FUNCTION_BLOCK FB_DirectControl EXTENDS FB_AsyncServiceResultClass
VAR
	_ipClient 	: I_ScsmClientClass;	
	_ipCtrl 	: I_AcsiCommonControllableDataClass;(* interface pointer to controllable data object *)

	_ctlVal		: U_AcsiCtlVal;
	_operTm 	: T_UtcTime;
	_origin		: ST_AcsiOriginator := ( orCat := E_AcsiOrCategory.StationControl, orIdent := [16#BE,16#CF,16#61,16#85] );
	_ctlNum		: USINT;
	_bTest 		: BOOL;
	_eCheck		: E_AcsiCheck := E_AcsiCheck.NoCheck; 	

	_nInvokeID 	: UDINT;
	_ipResult 	: I_AsyncServiceResultClass;

	_tmpCtlVal	: U_AcsiCtlVal;
	_bMxVal		: BOOL;
	state 		: UDINT;
END_VAR

METHOD APC : BOOL
VAR_INPUT
	ipClient 	: I_ScsmClientClass;	
	ipCtrl 		: I_AcsiCommonControllableDataClass;
	ctlVal		: REAL;
END_VAR
VAR_OUTPUT
	ipResult 	: I_AsyncServiceResultClass;
END_VAR
_tmpCtlVal.APC.f:= ctlVal;
APC:= Request(ipClient:=ipClient, ipCtrl:=ipCtrl, ctlVal:=_tmpCtlVal, bMxVal:=TRUE, ipResult=>ipResult);
END_METHOD

METHOD BAC : BOOL
VAR_INPUT
	ipClient 	: I_ScsmClientClass;	
	ipCtrl 		: I_AcsiCommonControllableDataClass;
	ctlVal		: E_AcsiTcmd;
END_VAR
VAR_OUTPUT
	ipResult 	: I_AsyncServiceResultClass;
END_VAR
_tmpCtlVal.BAC:= ctlVal;
BAC:= Request(ipClient:=ipClient, ipCtrl:=ipCtrl, ctlVal:=_tmpCtlVal, bMxVal:=TRUE, ipResult=>ipResult);
END_METHOD

METHOD BSC : BOOL
VAR_INPUT
	ipClient 	: I_ScsmClientClass;	
	ipCtrl 		: I_AcsiCommonControllableDataClass;
	ctlVal		: E_AcsiTcmd;
END_VAR
VAR_OUTPUT
	ipResult 	: I_AsyncServiceResultClass;
END_VAR
_tmpCtlVal.BSC:= ctlVal;
BSC:= Request(ipClient:=ipClient, ipCtrl:=ipCtrl, ctlVal:=_tmpCtlVal, bMxVal:=FALSE, ipResult=>ipResult);
END_METHOD

PROPERTY bTest : BOOL
SET
_bTest:= bTest;
END_SET
END_PROPERTY

METHOD Clear
VAR_INPUT
	ipReason : I_ServiceErrorClass;
END_VAR
IF SUPER^.IsBusy() THEN
	SUPER^.SetAborted(ipReason:=ipReason);
END_IF
state:= 0;
END_METHOD

METHOD DPC : BOOL
VAR_INPUT
	ipClient 	: I_ScsmClientClass;	
	ipCtrl 		: I_AcsiCommonControllableDataClass;
	ctlVal		: BOOL;
END_VAR
VAR_OUTPUT
	ipResult 	: I_AsyncServiceResultClass;
END_VAR
_tmpCtlVal.DPC:= ctlVal;
DPC:= Request(ipClient:=ipClient, ipCtrl:=ipCtrl, ctlVal:=_tmpCtlVal, bMxVal:=FALSE, ipResult=>ipResult);
END_METHOD

PROPERTY eCheck : E_AcsiCheck
SET
_eCheck:= eCheck;
END_SET
END_PROPERTY

METHOD ENC_Mod : BOOL
VAR_INPUT
	ipClient 	: I_ScsmClientClass;	
	ipCtrl 		: I_AcsiCommonControllableDataClass;
	ctlVal		: E_AcsiMod;
END_VAR
VAR_OUTPUT
	ipResult 	: I_AsyncServiceResultClass;
END_VAR
_tmpCtlVal.ENC.Mode:= ctlVal;
ENC_Mod:= Request(ipClient:=ipClient, ipCtrl:=ipCtrl, ctlVal:=_tmpCtlVal, bMxVal:=FALSE, ipResult=>ipResult);
END_METHOD

METHOD Execute : BOOL
CASE state OF
	0:RETURN;(* idle state *)

	(*--------------------- Verify status (optional) -----------------------------------*)
	1: (* Read control status information e.g.: "IEDLD1/CSWI1.ST.Pos" (stVal, q, t, ...) *)
		state:= SEL(_ipClient.GetDataValuesReq(ipData:=_ipCtrl, eFC:=SEL(_bMxVal, E_AcsiFc.ST_, E_AcsiFc.MX), hUser:=0, ipSink:=0, nInvokeID=>_nInvokeID, ipResult=>_ipResult), 100, 2); 
	2:
		IF _ipResult <> 0 THEN
			_ipResult.Execute();
			IF NOT _ipResult.IsBusy() THEN
				state:= SEL(_ipResult.IsCompleted(), 100, 10);
			END_IF
		END_IF
		
	(*--------------------- Verify config (optional) ------------------------------------*)
	10: (* Read control configuration e.g.: "IEDLD1/CSWI1.CF.Pos" (ctlModel, pulseConfig, ...) *)
		state:= SEL(_ipClient.GetDataValuesReq(ipData:=_ipCtrl, eFC:=E_AcsiFc.CF, hUser:=0, ipSink:=0, nInvokeID=>_nInvokeID, ipResult=>_ipResult), 100, 11); 
	11:
		IF _ipResult <> 0 THEN
			_ipResult.Execute();
			IF NOT _ipResult.IsBusy() THEN
				state:= SEL(_ipResult.IsCompleted(), 100, 12);
			END_IF
		END_IF

	12: (* Check ctlModel (optional) *)
		IF (_ipCtrl <> 0) AND_THEN (_ipCtrl.ipOper <> 0) AND_THEN (_ipCtrl.ipCtlModel <> 0) AND_THEN (_ipCtrl.ipCtlModel.eValue = E_AcsiCtlModels.DirectWithNormalSecurity) THEN
			state:= 20;
		ELSE(* fatal error *)
			state:= 90;
		END_IF
		
	(*--------------------- Operate ----------------------------------------------------*)
	20: (* Write "Oper" structure e.g.: "IEDLD1/CSWI1.CO.Pos.Oper" (ctlVal, operTm, origin, ctlNum, T, Test, Check, ...) *)
		_ctlNum:= _ctlNum + 1;(* create new ctlNum (optional) *)
		state:= SEL(_ipClient.ControlOperateReq(ipCtrl:=_ipCtrl, ctlVal:=_ctlVal, operTm:=_operTm, origin:=_origin, ctlNum:=_ctlNum, bTest:=_bTest, eCheck:=_eCheck, hUser:=0, ipSink:=0, nInvokeID=>_nInvokeID, ipResult=>_ipResult), 100, 21);  
	21:
		IF _ipResult <> 0 THEN
			_ipResult.Execute();
			IF NOT _ipResult.IsBusy() THEN
				state:= SEL(_ipResult.IsCompleted(), 100, 30);
			END_IF
		END_IF

	(*--------------------- Update status (optional) -----------------------------------*)
	30: (* Read control status information e.g.: "IEDLD1/CSWI1.ST.Pos" (stVal, q, t, ...) *)		
		state:= SEL(_ipClient.GetDataValuesReq(ipData:=_ipCtrl, eFC:=SEL(_bMxVal, E_AcsiFc.ST_, E_AcsiFc.MX), hUser:=0, ipSink:=0, nInvokeID=>_nInvokeID, ipResult=>_ipResult), 100, 31); 
	31:
		IF _ipResult <> 0 THEN
			_ipResult.Execute();
			IF NOT _ipResult.IsBusy() THEN
				state:= SEL(_ipResult.IsCompleted(), 100, 80);
			END_IF
		END_IF

	80: (* Completed *)
		state:= 0;
		SUPER^.SetCompleted();

	90: (* Fatal error *)
		state:= 0;
		SUPER^.SetFailedEx(stError:=TC_EVENTS.TcAcsiEventClass.AccessViolation);
		
	100: (* Failed or aborted *)
		state:= 0;
		SUPER^.CopyFrom(ipSource:=_ipResult);
END_CASE
Execute:= TRUE;
END_METHOD

METHOD INC : BOOL
VAR_INPUT
	ipClient 	: I_ScsmClientClass;	
	ipCtrl 		: I_AcsiCommonControllableDataClass;
	ctlVal		: DINT;
END_VAR
VAR_OUTPUT
	ipResult 	: I_AsyncServiceResultClass;
END_VAR
_tmpCtlVal.INC:= ctlVal;
INC:= Request(ipClient:=ipClient, ipCtrl:=ipCtrl, ctlVal:=_tmpCtlVal, bMxVal:=FALSE, ipResult=>ipResult);
END_METHOD

METHOD ISC : BOOL
VAR_INPUT
	ipClient 	: I_ScsmClientClass;	
	ipCtrl 		: I_AcsiCommonControllableDataClass;
	ctlVal		: SINT(-64..63);
END_VAR
VAR_OUTPUT
	ipResult 	: I_AsyncServiceResultClass;
END_VAR
_tmpCtlVal.ISC:= ctlVal;
ISC:= Request(ipClient:=ipClient, ipCtrl:=ipCtrl, ctlVal:=_tmpCtlVal, bMxVal:=FALSE, ipResult=>ipResult);
END_METHOD

PROPERTY operTm : T_UtcTime
SET
_operTm:= operTm;
END_SET
END_PROPERTY

PROPERTY origin : ST_AcsiOriginator
SET
_origin:= origin;
END_SET
END_PROPERTY

METHOD PRIVATE Request : BOOL
VAR_INPUT
	ipClient 	: I_ScsmClientClass;	
	ipCtrl 		: I_AcsiCommonControllableDataClass;
	ctlVal		: U_AcsiCtlVal;
	bMxVal		: BOOL;(* TRUE => status information is analogue value "mxVal", FALSE => status information is not analogue value "stVal" *)
END_VAR
VAR_OUTPUT
	ipResult : I_AsyncServiceResultClass := THIS^;
END_VAR
IF Request:=SUPER^.IsBusy() THEN
	RETURN;
END_IF

IF (ipClient = 0) OR (ipCtrl = 0) OR_ELSE (ipCtrl.ipOper = 0) OR_ELSE (ipCtrl.ipCtlModel = 0) THEN
	SUPER^.SetFailedEx(stError:=TC_EVENTS.TcAcsiEventClass.AccessViolation);
	RETURN;
END_IF 

_ipClient:= ipClient;
_ipCtrl:= ipCtrl;
_ctlVal:= ctlVal;
_bMxVal:= bMxVal;

SUPER^.SetBusy();
state:= 1;
Request:= TRUE;
END_METHOD

METHOD SPC : BOOL
VAR_INPUT
	ipClient 	: I_ScsmClientClass;	
	ipCtrl 		: I_AcsiCommonControllableDataClass;
	ctlVal		: BOOL;
END_VAR
VAR_OUTPUT
	ipResult 	: I_AsyncServiceResultClass;
END_VAR
_tmpCtlVal.SPC:= ctlVal;
SPC:= Request(ipClient:=ipClient, ipCtrl:=ipCtrl, ctlVal:=_tmpCtlVal, bMxVal:=FALSE, ipResult=>ipResult);
END_METHOD

END_FUNCTION_BLOCK
